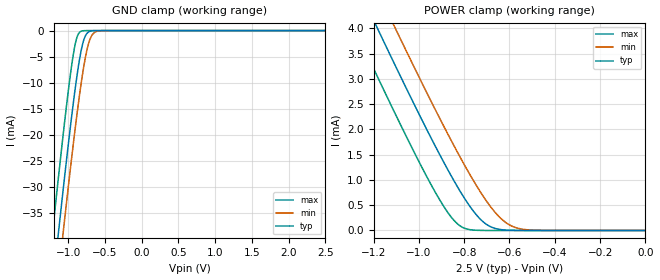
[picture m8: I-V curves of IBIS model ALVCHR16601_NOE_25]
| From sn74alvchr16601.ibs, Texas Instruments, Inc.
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[Model]   ALVCHR16601_NOE_25
Model_type  Input
Vinl=0.7
Vinh=1.7
| variable   typ   min   max
C_comp   2.07pF   1.76pF   2.32pF
[Temperature Range]   40   100   -40
| Ambient temperature   25   85   -40
[Voltage range]   2.5   2.3   2.7
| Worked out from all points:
|   GND clamp passes 1 mA (typ) near -0.77 V on its own axis
|   POWER clamp passes 1 mA (typ) near -0.85 V on its own axis
[GND Clamp]
| ALVCHR16601_NOE_25
|   Voltage   I(typ)   I(min)   I(max)
-2.5V     -228.3mA   -236mA     -218.7mA
-1.23V    -51.64mA   -59.93mA   -41.01mA
-1.2V     -47.65mA   -55.95mA   -37mA
-1.13V    -38.46mA   -46.75mA   -27.8mA
-1.07V    -30.74mA   -39mA      -20.15mA
-925mV    -13.31mA   -21.13mA   -4.126mA
-880mV    -8.615mA   -16.01mA   -1.264mA
-830mV    -4.285mA   -10.76mA   -171.7uA
-780mV    -1.473mA   -6.233mA   -17.16uA
-720mV    -242.7uA   -2.356mA   -1.024uA
-600mV    -3.836uA   -109.3uA   -3.611nA
2.5V      4.713pA    7.579pA    4.389pA
[POWER Clamp]
| ALVCHR16601_NOE_25
|   Voltage   I(typ)   I(min)   I(max)
-2.5V     16.88mA    17.58mA    15.98mA
-1.3V     5.111mA    5.849mA    4.158mA
-1.255V   4.681mA    5.42mA     3.727mA
-1.18V    3.971mA    4.711mA    3.015mA
-1.11V    3.316mA    4.055mA    2.36mA
-940mV    1.776mA    2.501mA    856.4uA
-845mV    982.9uA    1.676mA    200.1uA
-795mV    611.2uA    1.266mA    38.41uA
-725mV    207uA      738.7uA    1.527uA
-625mV    11.21uA    186.8uA    11.91nA
-510mV    181.6nA    9.688uA    51.12pA
-31.15fV  4.712pA    6.41pA     4.886pA
